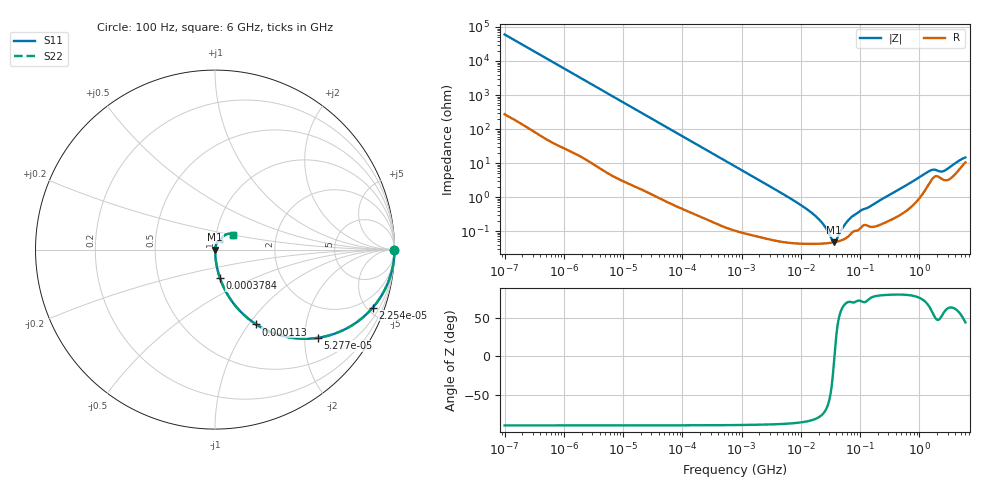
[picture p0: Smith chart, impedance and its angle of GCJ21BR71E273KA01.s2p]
!Murata Part Number: GCJ21BR71E273KA01
!These Parameters are Measured in Series Mode Connection
!Data Generated on Mar 13, 2026
!  o--ll--o
!Port1  Port2
!  o------o
!Operation Temp=25[degC], DC Bias Voltage=0[V]
!Freq. Start=100[Hz] Stop=6[GHz] 401[Steps]
# Hz S RI R 50
!Freq.(Hz) S11(Real) S11(Imag) S21(Real) S21(Imag) S12(Real) S12(Imag) S22(Real) S22(Imag)
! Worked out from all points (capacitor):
!   401 points, 100 Hz to 6 GHz, reference 50 ohm
!   read as one part in series: C = 26.4 nF near 109 Hz
!   lowest |Z| = 47.3 mohm at 36.42 MHz (marker M1)
!   series resonance near 36.94 MHz, so ESL is about 700 pH
!   S11 on the Smith chart (normalised r, x): 100 Hz: open; 22.54 kHz: 1.03, -5.42; 52.77 kHz: 1.01, -2.32; 113 kHz: 1.01, -1.09; 378.4 kHz: 1.00, -0.33; 6 GHz: 1.21, +0.20
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100  1 -0.00166  1.03e-05 0.00166  1.03e-05 0.00166  1 -0.00166
2008  0.9987 -0.0331  0.00126 0.0331  0.00126 0.0331  0.9987 -0.0331
7695  0.9837 -0.1243  0.0163 0.1243  0.0163 0.1243  0.9837 -0.1243
22537  0.8788 -0.3236  0.1212 0.3236  0.1212 0.3236  0.8788 -0.3236
40335  0.6962 -0.4568  0.3038 0.4568  0.3038 0.4568  0.6962 -0.4568
52766  0.5737 -0.4913  0.4263 0.4913  0.4263 0.4913  0.5737 -0.4913
112960  0.2301 -0.4172  0.7699 0.4172  0.7699 0.4172  0.2301 -0.4172
193316  0.0942 -0.2879  0.9058 0.2879  0.9058 0.2879  0.0942 -0.2879
378399  0.0275 -0.1586  0.9725 0.1586  0.9725 0.1586  0.0275 -0.1586
774597  0.00737 -0.0794  0.9926 0.0794  0.9926 0.0794  0.00737 -0.0794
6353432  0.000544 -0.00959  0.9995 0.00959  0.9995 0.00959  0.000544 -0.00959
1.555665e7  0.000432 -0.00333  0.9996 0.00333  0.9996 0.00333  0.000432 -0.00333
2.327686e7  0.000432 -0.00163  0.9996 0.00163  0.9996 0.00163  0.000432 -0.00163
3.330331e7  0.000458 -0.000355  0.9995 0.000355  0.9995 0.000355  0.000458 -0.000355
3.64232e7  0.000471 -4.77e-05  0.9995 4.77e-05  0.9995 4.77e-05  0.000471 -4.77e-05
3.983537e7  0.000486 0.00026  0.9995 -0.00026  0.9995 -0.00026  0.000486 0.00026
5.449875e7  0.000588 0.00138  0.9994 -0.00138  0.9994 -0.00138  0.000588 0.00138
7.129496e7  0.000867 0.00243  0.9991 -0.00243  0.9991 -0.00243  0.000867 0.00243
3.124326e8  0.00215 0.0114  0.9978 -0.0114  0.9978 -0.0114  0.00215 0.0114
1.431855e9  0.0251 0.0494  0.9749 -0.0494  0.9749 -0.0494  0.0251 0.0494
2.562649e9  0.0333 0.0452  0.9667 -0.0452  0.9667 -0.0452  0.0333 0.0452
6e9  0.1024 0.0824  0.8976 -0.0824  0.8976 -0.0824  0.1024 0.0824
